| IBIS file stm32l4r9_s9_ufbga144.ibs
[IBIS ver]   4.2
[File name]   stm32l4r9_s9_ufbga144.ibs
[File Rev]   1.0
[Date]   01-6-2017
[Source]   Data Created at STMicroelectronics
[Notes]   File originated from ELDO simulations.
[Disclaimer]  This information is for modeling purpose only and is
   not guaranted.
   The information is subject to change without notice.
[Copyright]   Copyright 2017 STMicroelectronics Inc.
|   Component stm32l4r9_s9_ufbga144
[Component] stm32l4r9_s9_ufbga144
[Manufacturer] STMicroelectronics
[Package]
| variable   typ   min   max
R_pkg   0.0   0.0   0.0
L_pkg   0.0H   0.0H   0.0H
C_pkg   0.0F   0.0F   0.0F
[Pin]  signal_name   model_name   R_pin   L_pin   C_pin
A1 VSS gnd
A10 PA14 io8prog2m25m50m120m_sudq_ft
A11 VDD power
A12 VSS gnd
A2 PE0 io8prog2m25m50m120m_sudq_ft
A3 PB9 io8prog2m25m50m120m_sudq_i2c_ft
A4 PH3-BOOT0 io8prog2m25m50m120m_sudq_ft
A5 PB4 io8prog2m25m50m120m_sudq_i2c_ft
A6 VDDIO2 power
A7 VSS gnd
A8 PD3 io8prog2m25m50m120m_sudq_ft
A9 PC11 io8prog2m25m50m120m_sudq_ft
B1 VBAT power
B10 PA13 io8prog2m25m50m120m_sudq_ft
B11 PA12 io8usblsfs_otg2
B12 PA11 io8usblsfs_otg2
B2 VDD power
B3 PE3 io8prog2m25m50m120m_sudq_ft
B4 PB8 io8prog2m25m50m120m_sudq_i2c_ft
B5 PB5 io8prog2m25m50m120m_sudq_ft
B6 PB3 io8prog2m25m50m120m_sudq_ft
B7 PD6 io8prog2m25m50m120m_sudq_ft
B8 PD1 io8prog2m25m50m120m_sudq_ft
B9 PA15 io8prog2m25m50m120m_sudq_ft
C1 VSS gnd
C10 PA10 io8usb_id_otg20_lcd4_ft_ms
C11 VDDUSB power
C12 PC9 io8prog2m25m50m120m_sudq_ft
C2 PE5 io8prog2m25m50m120m_sudq_ft
C3 PE2 io8prog2m25m50m120m_sudq_ft
C4 PE1 io8prog2m25m50m120m_sudq_ft
C5 PB7 io8prog2m25m50m120m_sudq_i2c_ft
C6 PG13 io8prog2m25m50m120m_sudq_i2c_ft
C7 PD4 io8prog2m25m50m120m_sudq_ft
C8 PD0 io8prog2m25m50m120m_sudq_ft
C9 PC10 io8prog2m25m50m120m_sudq_ft
D1 PC14-OSC32_IN io8prog2m25m50m120m_sudq_ft
D10 PA9 power
D11 PA8 io8prog2m25m50m120m_sudq_ft
D12 PC6 io8prog2m25m50m120m_sudq_ft
D2 PC15-OSC32_OUT io8prog2m25m50m120m_sudq_ft
D3 PE4 io8prog2m25m50m120m_sudq_ft
D4 PE6 io8prog2m25m50m120m_sudq_ft
D5 PB6 io8prog2m25m50m120m_sudq_i2c_ft
D6 PG12 io8prog2m25m50m120m_sudq_ft
D7 PD5 io8prog2m25m50m120m_sudq_ft
D8 PD2 io8prog2m25m50m120m_sudq_ft
D9 PC12 io8prog2m25m50m120m_sudq_ft
E1 PF2 io8prog2m25m50m120m_sudq_ft
E10 PC8 io8prog2m25m50m120m_sudq_ft
E11 PG7 io8prog2m25m50m120m_sudq_i2c_ft
E12 VDDIO2 power
E2 PF1 io8prog2m25m50m120m_sudq_i2c_ft
E3 PF0 io8prog2m25m50m120m_sudq_i2c_ft
E4 PC13 io8prog2m25m50m120m_sudq_ft
E5 PF3 io8prog2m25m50m120m_sudq_ft
E6 PG10 io8prog2m25m50m120m_sudq_ft
E7 PD7 io8prog2m25m50m120m_sudq_ft
E8 PG8 io8prog2m25m50m120m_sudq_i2c_ft
E9 PC7 io8prog2m25m50m120m_sudq_ft
F1 PF8 io8prog2m25m50m120m_sudq_ft
F10 PG4 io8prog2m25m50m120m_sudq_ft
F11 VSS gnd
F12 PG2 io8prog2m25m50m120m_sudq_ft
F2 PF6 io8prog2m25m50m120m_sudq_ft
F3 PF4 io8prog2m25m50m120m_sudq_ft
F4 PF5 io8prog2m25m50m120m_sudq_ft
F5 PF7 io8prog2m25m50m120m_sudq_ft
F6 PG9 io8prog2m25m50m120m_sudq_ft
F7 PG3 io8prog2m25m50m120m_sudq_ft
F8 PG5 io8prog2m25m50m120m_sudq_ft
F9 PG6 io8prog2m25m50m120m_sudq_ft
G1 VDD power
G10 PD13 io8prog2m25m50m120m_sudq_ft
G11 PD11 io8prog2m25m50m120m_sudq_ft
G12 VDD power
G2 VSS gnd
G3 PF10 io8prog2m25m50m120m_sudq_ft
G4 PF9 io8prog2m25m50m120m_sudq_ft
G5 PF12 io8prog2m25m50m120m_sudq_ft
G6 PE7 io8prog2m25m50m120m_sudq_ft
G7 PD15 io8prog2m25m50m120m_sudq_ft
G8 PD14 io8prog2m25m50m120m_sudq_ft
G9 PD12 io8prog2m25m50m120m_sudq_ft
H1 PH0-OSC_IN io8prog2m25m50m120m_sudq_ft
H10 PD8 io8prog2m25m50m120m_sudq_ft
H11 DSI_D1P NC
H12 DSI_D1N NC
H2 PH1-OSC_OUT io8prog2m25m50m120m_sudq_ft
H3 PC0 io8prog2m25m50m120m_sudq_i2c_ft
H4 PC2 io8prog2m25m50m120m_sudq_ft
H5 PB2 io8prog2m25m50m120m_sudq_ft
H6 PF15 io8prog2m25m50m120m_sudq_i2c_ft
H7 PE11 io8prog2m25m50m120m_sudq_ft
H8 PD10 io8prog2m25m50m120m_sudq_ft
H9 PD9 io8prog2m25m50m120m_sudq_ft
J1 NRST ioreset_ft_v33
J10 VSSDSI gnd
J11 DSI_CKP NC
J12 DSI_CKN NC
J2 PC1 io8prog2m25m50m120m_sudq_i2c_ft
J3 PC3 io8prog2m25m50m120m_sudq_ft
J4 PA6 io8prog2m25m50m120m_sudq_ft
J5 PB1 io8prog2m25m50m120m_sudq_ft
J6 PF13 io8prog2m25m50m120m_sudq_ft
J7 PE9 io8prog2m25m50m120m_sudq_ft
J8 PE13 io8prog2m25m50m120m_sudq_ft
J9 PB15 io8prog2m25m50m120m_sudq_ft
K1 VSSA/VREF- gnd
K10 PB14 io8prog2m25m50m120m_sudq_i2c_ft
K11 DSI_D0P NC
K12 DSI_D0N NC
K2 VREF+ power
K3 PA0 io8prog2m25m50m120m_sudq_ft
K4 PA4 io8prog2m25m50m120m_sudq_ft
K5 PC5 io8prog2m25m50m120m_sudq_ft
K6 PF11 io8prog2m25m50m120m_sudq_ft
K7 PE8 io8prog2m25m50m120m_sudq_ft
K8 PE15 io8prog2m25m50m120m_sudq_ft
K9 PB11 io8prog2m25m50m120m_sudq_i2c_ft
L1 VDDA power
L10 PB12 io8prog2m25m50m120m_sudq_ft
L11 VDD power
L12 VCAPDSI power
L2 PA1 io8prog2m25m50m120m_sudq_ft
L3 PA2 io8prog2m25m50m120m_sudq_ft
L4 PA5 io8prog2m25m50m120m_sudq_ft
L5 PC4 io8prog2m25m50m120m_sudq_ft
L6 VSS gnd
L7 PG0 io8prog2m25m50m120m_sudq_ft
L8 PE10 io8prog2m25m50m120m_sudq_ft
L9 PB10 io8prog2m25m50m120m_sudq_i2c_ft
M1 VSS gnd
M10 PE14 io8prog2m25m50m120m_sudq_ft
M11 PB13 io8prog2m25m50m120m_sudq_i2c_ft
M12 VSS gnd
M2 VDD power
M3 PA3 io8prog2m25m50m120m_sudq_ft
M4 PA7 io8prog2m25m50m120m_sudq_i2c_ft
M5 PB0 io8prog2m25m50m120m_sudq_ft
M6 VDD power
M7 PF14 io8prog2m25m50m120m_sudq_i2c_ft
M8 PG1 io8prog2m25m50m120m_sudq_ft
M9 PE12 io8prog2m25m50m120m_sudq_ft
[Diff Pin]   inv_pin   vdiff   tdelay_typ  tdelay_min  tdelay_max
B11 B12 200mV   NA   NA   NA
[Model Selector] io8prog2m25m50m120m_sudq_ft
io8p00_sudq_ft_pd_lv  "SPEED00, PD=40kOhm - 1P8V"
io8p00_sudq_ft_pu_lv  "SPEED00, PU=40kOhm - 1P8V"
io8p00_sudq_ft_lv  "SPEED00 - 1P8V"
io8p00_sudq_ft_pd  "SPEED00, PD=40kOhm - 3P3V"
io8p00_sudq_ft_pu  "SPEED00, PU=40kOhm - 3P3V"
io8p00_sudq_ft  "SPEED00 - 3P3V"
io8p01_sudq_ft_pd_lv  "SPEED01, PD=40kOhm - 1P8V"
io8p01_sudq_ft_pu_lv  "SPEED01, PU=40kOhm - 1P8V"
io8p01_sudq_ft_lv  "SPEED01 - 1P8V"
io8p01_sudq_ft_pd  "SPEED01, PD=40kOhm - 3P3V"
io8p01_sudq_ft_pu  "SPEED01, PU=40kOhm - 3P3V"
io8p01_sudq_ft  "SPEED01 - 3P3V"
io8p10_sudq_ft_pd_lv  "SPEED10, PD=40kOhm - 1P8V"
io8p10_sudq_ft_pu_lv  "SPEED10, PU=40kOhm - 1P8V"
io8p10_sudq_ft_lv  "SPEED10 - 1P8V"
io8p10_sudq_ft_pd  "SPEED10, PD=40kOhm - 3P3V"
io8p10_sudq_ft_pu  "SPEED10, PU=40kOhm - 3P3V"
io8p10_sudq_ft  "SPEED10 - 3P3V"
io8p11_sudq_ft_pd_lv  "SPEED11, PD=40kOhm - 1P8V"
io8p11_sudq_ft_pu_lv  "SPEED11, PU=40kOhm - 1P8V"
io8p11_sudq_ft_lv  "SPEED11 - 1P8V"
io8p11_sudq_ft_pd  "SPEED11, PD=40kOhm - 3P3V"
io8p11_sudq_ft_pu  "SPEED11, PU=40kOhm - 3P3V"
io8p11_sudq_ft  "SPEED11 - 3P3V"
[Model Selector] io8prog2m25m50m120m_sudq_i2c_ft
io8prog_1v8_i2c_pd  "5V Tol GPIO 1.8V range i2c functionality with pull down"
io8prog_1v8_i2c_pu  "5V Tol GPIO 1.8V range i2c functionality with pull up"
io8prog_1v8_i2c  "5V Tol GPIO 1.8V range i2c functionality"
io8prog_3v3_i2c_pd  "5V Tol GPIO 3.3V range i2c functionality with pull down"
io8prog_3v3_i2c_pu  "5V Tol GPIO 3.3V range i2c functionality with pull up"
io8prog_3v3_i2c  "5V Tol GPIO 3.3V range i2c functionality"
io8prog_1v8_pd_00  "5V Tol GPIO 1.8V range with pd speed 00"
io8prog_1v8_pu_00  "5V Tol GPIO 1.8V range with pu speed 00"
io8prog_1v8_00  "5V Tol GPIO 1.8V range speed 00"
io8prog_3v3_pd_00  "5V Tol GPIO 3.3V range with pd speed 00"
io8prog_3v3_pu_00  "5V Tol GPIO 3.3V range with pu speed 00"
io8prog_3v3_00  "5V Tol GPIO 3.3V range speed 00"
io8prog_1v8_pd_01  "5V Tol GPIO 1.8V range with pd speed 01"
io8prog_1v8_pu_01  "5V Tol GPIO 1.8V range with pu speed 01"
io8prog_1v8_01  "5V Tol GPIO 1.8V range speed 01"
io8prog_3v3_pd_01  "5V Tol GPIO 3.3V range with pd speed 01"
io8prog_3v3_pu_01  "5V Tol GPIO 3.3V range with pu speed 01"
io8prog_3v3_01  "5V Tol GPIO 3.3V range speed 01"
io8prog_1v8_pd_10  "5V Tol GPIO 1.8V range with pd speed 10"
io8prog_1v8_pu_10  "5V Tol GPIO 1.8V range with pu speed 10"
io8prog_1v8_10  "5V Tol GPIO 1.8V range speed 10"
io8prog_3v3_pd_10  "5V Tol GPIO 3.3V range with pd speed 10"
io8prog_3v3_pu_10  "5V Tol GPIO 3.3V range with pu speed 10"
io8prog_3v3_10  "5V Tol GPIO 3.3V range speed 10"
io8prog_1v8_pd_11  "5V Tol GPIO 1.8V range with pd speed 11"
io8prog_1v8_pu_11  "5V Tol GPIO 1.8V range with pu speed 11"
io8prog_1v8_11  "5V Tol GPIO 1.8V range speed 11"
io8prog_3v3_pd_11  "5V Tol GPIO 3.3V range with pd speed 11"
io8prog_3v3_pu_11  "5V Tol GPIO 3.3V range with pu speed 11"
io8prog_3v3_11  "5V Tol GPIO 3.3V range speed 11"
[Model Selector] io8usb_id_otg20_lcd4_ft_ms
io8usbid_1v8_id_pu  "ID 1V8 range with pull up"
io8usbid_3v3_id_pu  "ID 3V3 range with pull up"
io8usbid_1v8_id  "ID 1V8 range"
io8usbid_3v3_id  "ID 3V3 range"
io8usbid_1v8_pd_00  "GPIO 1.8V range with pd speed 00"
io8usbid_1v8_pu_00  "GPIO 1.8V range with pu speed 00"
io8usbid_1v8_00  "GPIO 1.8V range speed 00"
io8usbid_3v3_pd_00  "GPIO 3.3V range with pd speed 00"
io8usbid_3v3_pu_00  "GPIO 3.3V range with pu speed 00"
io8usbid_3v3_00  "GPIO 3.3V range speed 00"
io8usbid_1v8_pd_01  "GPIO 1.8V range with pd speed 01"
io8usbid_1v8_pu_01  "GPIO 1.8V range with pu speed 01"
io8usbid_1v8_01  "GPIO 1.8V range speed 01"
io8usbid_3v3_pd_01  "GPIO 3.3V range with pd speed 01"
io8usbid_3v3_pu_01  "GPIO 3.3V range with pu speed 01"
io8usbid_3v3_01  "GPIO 3.3V range speed 01"
io8usbid_1v8_pd_10  "GPIO 1.8V range with pd speed 10"
io8usbid_1v8_pu_10  "GPIO 1.8V range with pu speed 10"
io8usbid_1v8_10  "GPIO 1.8V range speed 10"
io8usbid_3v3_pd_10  "GPIO 3.3V range with pd speed 10"
io8usbid_3v3_pu_10  "GPIO 3.3V range with pu speed 10"
io8usbid_3v3_10  "GPIO 3.3V range speed 10"
io8usbid_1v8_pd_11  "GPIO 1.8V range with pd speed 11"
io8usbid_1v8_pu_11  "GPIO 1.8V range with pu speed 11"
io8usbid_1v8_11  "GPIO 1.8V range speed 11"
io8usbid_3v3_pd_11  "GPIO 3.3V range with pd speed 11"
io8usbid_3v3_pu_11  "GPIO 3.3V range with pu speed 11"
io8usbid_3v3_11  "GPIO 3.3V range speed 11"
[Model Selector] io8usblsfs_otg2
usb_ls_pd  "USB Low Speed mode - Pull Down"
usb_ls_pu2  "USB Low Speed mode - Pull up 2"
usb_ls_pu  "USB Low Speed mode - Pull up"
usb_fs  "USB Low Speed mode"
usb_fs_pd  "USB Full Speed mode - Pull Down"
usb_fs_pu2  "USB Full Speed mode - Pull up 2"
usb_fs_pu  "USB Full Speed mode - Pull up"
[Model Selector] ioreset_ft_v33
ioreset_1v2_pu  "RESET 1.2V range with PU"
ioreset_1v2  "RESET 1.2V range"
ioreset_1v8_pu  "RESET 1.8V range with PU"
ioreset_1v8  "RESET 1.8V range"
ioreset_3v3_pu  "RESET 3.3V range with PU"
ioreset_3v3  "RESET 3.3V range"
| Models and submodels in the file (95): io8p00_sudq_ft_pd_lv (I/O), io8p00_sudq_ft_pu_lv (I/O), io8p00_sudq_ft_lv (I/O), io8p00_sudq_ft_pd (I/O), io8p00_sudq_ft_pu (I/O), io8p00_sudq_ft (I/O), io8p01_sudq_ft_pd_lv (I/O), io8p01_sudq_ft_pu_lv (I/O), io8p01_sudq_ft_lv (I/O), io8p01_sudq_ft_pd (I/O), io8p01_sudq_ft_pu (I/O), io8p01_sudq_ft (I/O), io8p10_sudq_ft_pd_lv (I/O), io8p10_sudq_ft_pu_lv (I/O), io8p10_sudq_ft_lv (I/O), io8p10_sudq_ft_pd (I/O), io8p10_sudq_ft_pu (I/O), io8p10_sudq_ft (I/O), io8p11_sudq_ft_pd_lv (I/O), io8p11_sudq_ft_pu_lv (I/O), io8p11_sudq_ft_lv (I/O), io8p11_sudq_ft_pd (I/O), io8p11_sudq_ft_pu (I/O), io8p11_sudq_ft (I/O), io8prog_1v8_i2c_pd (I/O), io8prog_1v8_i2c_pu (I/O), io8prog_1v8_i2c (I/O), io8prog_3v3_i2c_pd (I/O), io8prog_3v3_i2c_pu (I/O), io8prog_3v3_i2c (I/O), io8prog_1v8_pd_00 (I/O), io8prog_1v8_pu_00 (I/O), io8prog_1v8_00 (I/O), io8prog_3v3_pd_00 (I/O), io8prog_3v3_pu_00 (I/O), io8prog_3v3_00 (I/O), io8prog_1v8_pd_01 (I/O), io8prog_1v8_pu_01 (I/O), io8prog_1v8_01 (I/O), io8prog_3v3_pd_01 (I/O), io8prog_3v3_pu_01 (I/O), io8prog_3v3_01 (I/O), io8prog_1v8_pd_10 (I/O), io8prog_1v8_pu_10 (I/O), io8prog_1v8_10 (I/O), io8prog_3v3_pd_10 (I/O), io8prog_3v3_pu_10 (I/O), io8prog_3v3_10 (I/O), io8prog_1v8_pd_11 (I/O), io8prog_1v8_pu_11 (I/O), io8prog_1v8_11 (I/O), io8prog_3v3_pd_11 (I/O), io8prog_3v3_pu_11 (I/O), io8prog_3v3_11 (I/O), io8usbid_1v8_id_pu (Input), io8usbid_3v3_id_pu (Input), io8usbid_1v8_id (Input), io8usbid_3v3_id (Input), io8usbid_1v8_pd_00 (I/O), io8usbid_1v8_pu_00 (I/O), io8usbid_1v8_00 (I/O), io8usbid_3v3_pd_00 (I/O), io8usbid_3v3_pu_00 (I/O), io8usbid_3v3_00 (I/O), io8usbid_1v8_pd_01 (I/O), io8usbid_1v8_pu_01 (I/O), io8usbid_1v8_01 (I/O), io8usbid_3v3_pd_01 (I/O), io8usbid_3v3_pu_01 (I/O), io8usbid_3v3_01 (I/O), io8usbid_1v8_pd_10 (I/O), io8usbid_1v8_pu_10 (I/O), io8usbid_1v8_10 (I/O), io8usbid_3v3_pd_10 (I/O), io8usbid_3v3_pu_10 (I/O), io8usbid_3v3_10 (I/O), io8usbid_1v8_pd_11 (I/O), io8usbid_1v8_pu_11 (I/O), io8usbid_1v8_11 (I/O), io8usbid_3v3_pd_11 (I/O)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
